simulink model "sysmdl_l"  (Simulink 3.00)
settings: Solver=ode45  SolverMode=SingleTasking  StartTime=0.0  StopTime=10.0  RelTol=1e-3  AbsTol=1e-6
undefined symbols (not defined in the file or in its folder): pow

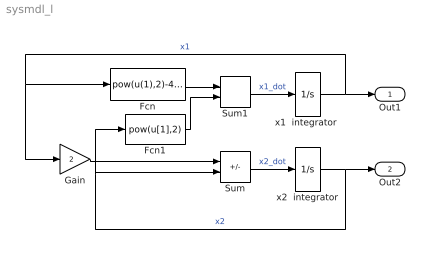
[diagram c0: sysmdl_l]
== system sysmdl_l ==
  Fcn : Fcn  Expr=pow(u(1),2)-4.0
  Fcn1 : Fcn  Expr=pow(u[1],2)
  Gain : Gain  Gain=2  SaturateOnIntegerOverflow=on
  Sum : Sum  Inputs=+-  SaturateOnIntegerOverflow=on
  Sum1 : Sum  Inputs=++  SaturateOnIntegerOverflow=on
  "x1  integrator " : Integrator  ExternalReset=none  InitialConditionSource=internal  InitialCondition=0  LimitOutput=off  UpperSaturationLimit=inf  LowerSaturationLimit=-inf  ShowSaturationPort=off  ShowStatePort=off  AbsoluteTolerance=auto
  x2  integrator : Integrator  ExternalReset=none  InitialConditionSource=internal  InitialCondition=0  LimitOutput=off  UpperSaturationLimit=inf  LowerSaturationLimit=-inf  ShowSaturationPort=off  ShowStatePort=off  AbsoluteTolerance=auto
  Out1 : Outport  Port=1
  Out2 : Outport  Port=2
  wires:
  Gain/1 -> Sum/1
  Sum/1 -> x2  integrator/1  "x2_dot"
  Fcn/1 -> Sum1/1
  Sum1/1 -> "x1  integrator "/1  "x1_dot"
  "x1  integrator "/1 -> Gain/1, Fcn/1, Out1/1  "x1"
  x2  integrator/1 -> Sum/2, Fcn1/1, Out2/1  "x2"
  Fcn1/1 -> Sum1/2
